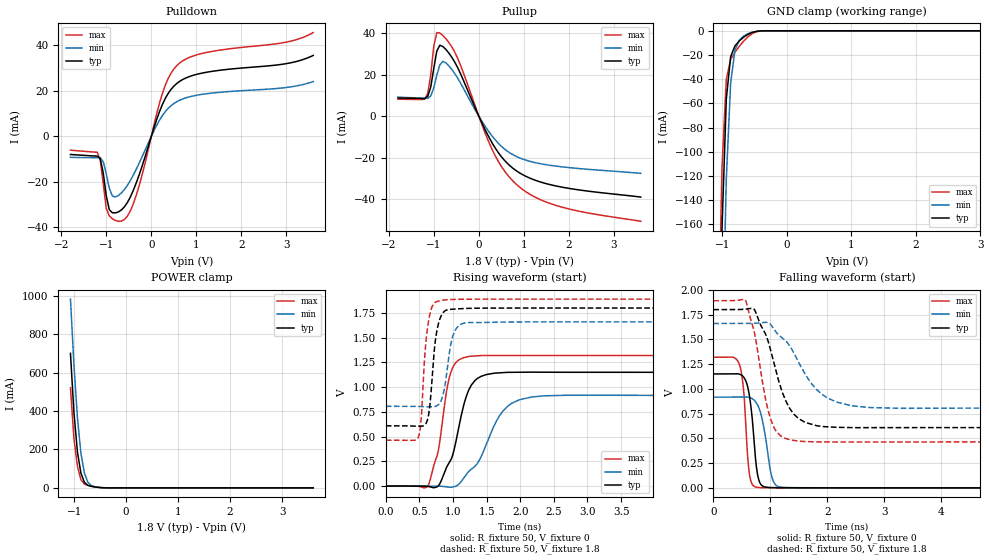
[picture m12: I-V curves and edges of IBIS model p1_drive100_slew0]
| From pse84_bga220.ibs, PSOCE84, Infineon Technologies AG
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[Model] p1_drive100_slew0
Model_type I/O
Polarity  Non-Inverting
Enable   Active-High
Vinl  =  0.54
Vinh  =  1.26
Vmeas =  0.9
Cref  =  15pF
| Capacitance   typ   min   max
C_comp   1.187163e-12   1.148471e-12   1.233738e-12
| Variables   typ   min   max
[GND Clamp Reference]   0   0   0
[POWER Clamp Reference]   1.8   1.66   1.89
[Pulldown Reference]   0   0   0
[Pullup Reference]   1.8   1.66   1.89
[Temperature Range]   25   125   -40
[Voltage Range]   1.8   1.66   1.89
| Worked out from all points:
|   slope of the pulldown table from 0 to 0.27 V, typ, clamps not added: 18 ohm
|   slope of the pullup table from 0 to 0.27 V, typ, clamps not added: 22.7 ohm
|   GND clamp passes 1 mA (typ) near -0.51 V on its own axis
|   POWER clamp passes 1 mA (typ) near -0.47 V on its own axis
|   rising waveform, R_fixture 50, V_fixture 0: 20-80 % time 266ps typ, 419ps min, 189ps max; typ from 0 V to 1.15 V
|   rising waveform, R_fixture 50, V_fixture 1.8: 20-80 % time 97.2ps typ, 117ps min, 87.9ps max; typ from 0.609 V to 1.8 V
|   falling waveform, R_fixture 50, V_fixture 0: 20-80 % time 116ps typ, 158ps min, 91.1ps max; typ from 1.15 V to 0 V
|   falling waveform, R_fixture 50, V_fixture 1.8: 20-80 % time 392ps typ, 582ps min, 272ps max; typ from 1.8 V to 0.609 V
[GND Clamp]
| Voltage   I(typ)   I(min)   I(max)
-1.137V   -618.8mA   -753.3mA   -532.4mA
-1.07V    -360.9mA   -497.6mA   -281.1mA
-1.003V   -163.7mA   -277.5mA   -113mA
-936.6mV  -56.21mA   -122.2mA   -40.06mA
-869.7mV  -21.33mA   -43.29mA   -23.66mA
-802.8mV  -12.5mA    -15.96mA   -17.71mA
-735.9mV  -8.345mA   -7.674mA   -12.88mA
-669mV    -5.267mA   -4.349mA   -8.574mA
-535.2mV  -1.314mA   -1.207mA   -2.328mA
-401.4mV  -73.55uA   -132.2uA   -119.3uA
3.6V      0A         0A         0A
[POWER Clamp]
| Voltage   I(typ)   I(min)   I(max)
-1.07V    700.8mA    983.4mA    521.5mA
-1.003V   391.6mA    640.4mA    255.8mA
-936.6mV  187.6mA    365.2mA    112.5mA
-869.7mV  77.29mA    181mA      42.73mA
-802.8mV  28.91mA    77.52mA    19.98mA
-735.9mV  13.13mA    29.19mA    13.35mA
-669mV    7.755mA    11.55mA    8.955mA
-535.2mV  2.356mA    2.862mA    2.667mA
-334.5mV  34.33uA    127.4uA    15.58uA
3.6V      0A         0A         0A
[Pullup]
| Voltage   I(typ)   I(min)   I(max)
-1.8V     8.819mA    9.225mA    8.256mA
-1.204V   8.594mA    8.734mA    8.362mA
-1.07V    14.25mA    9.887mA    20.21mA
-1.003V   23.19mA    13.79mA    33.91mA
-936.6mV  31.46mA    19.78mA    40.38mA
-869.7mV  34.26mA    24.82mA    40.18mA
-735.9mV  32.26mA    25.83mA    37.45mA
-468.3mV  23.29mA    18.27mA    27.8mA
310.3mV   -13.41mA   -9.935mA   -16.71mA
806.9mV   -25.84mA   -19.05mA   -32.25mA
1.738V    -33.65mA   -24.05mA   -43.07mA
3.6V      -38.9mA    -27.47mA   -50.57mA
[Pulldown]
| Voltage   I(typ)   I(min)   I(max)
-1.8V     -8.09mA    -9.336mA   -6.18mA
-1.204V   -8.819mA   -9.493mA   -7.128mA
-1.137V   -9.825mA   -9.491mA   -10.67mA
-1.003V   -26.32mA   -16.67mA   -31.9mA
-936.6mV  -32.37mA   -22.89mA   -35.09mA
-869.7mV  -33.73mA   -26.29mA   -36.32mA
-669mV    -32.52mA   -25.02mA   -37.41mA
-401.4mV  -23.83mA   -17.14mA   -29.77mA
248.3mV   14.08mA    9.149mA    19.02mA
558.6mV   23.07mA    15.08mA    30.9mA
1.117V    27.69mA    18.36mA    36.34mA
3.6V      35.52mA    24.01mA    45.58mA
[Ramp]
dV/dt_r   0.690092/0.265717n  0.54975/0.418773n  0.791747/0.1894n
dV/dt_f   0.714838/0.391602n  0.512302/0.581669n  0.855898/0.272071n
R_load = 50
[Rising Waveform]
R_fixture = 50
V_fixture = 0
V_fixture_min = 0
V_fixture_max = 0
| Time   V(typ)   V(min)   V(max)
0s        14.93nV    1.041uV    5.447nV
609.9ps   -2.759mV   823.6nV    -10.2mV
786.7ps   6.51mV     -1.184mV   381.1mV
898.1ps   181.7mV    -7.774mV   938mV
983.7ps   291.3mV    -11.34mV   1.182V
1.203ns   919.2mV    123.2mV    1.305V
1.395ns   1.101V     267.5mV    1.319V
1.81ns    1.15V      805.9mV    1.32V
2.678ns   1.15V      917.8mV    1.319V
50ns      1.15V      916.3mV    1.32V
[Rising Waveform]
R_fixture = 50
V_fixture = 1.8
V_fixture_min = 1.66
V_fixture_max = 1.89
| Time   V(typ)   V(min)   V(max)
0s        608.6mV    806.2mV    463.5mV
486.4ps   605mV      804.5mV    500.3mV
525ps     605mV      803.2mV    669.8mV
600.4ps   635.9mV    801.8mV    1.487V
765.6ps   1.592V     813.1mV    1.867V
862.2ps   1.761V     953.2mV    1.881V
967.8ps   1.787V     1.437V     1.886V
1.147ns   1.795V     1.644V     1.889V
1.907ns   1.8V       1.659V     1.89V
50ns      1.8V       1.66V      1.89V
[Falling Waveform]
R_fixture = 50
V_fixture = 0
V_fixture_min = 0
V_fixture_max = 0
| Time   V(typ)   V(min)   V(max)
0s        1.15V      916.3mV    1.32V
448.9ps   1.149V     916.6mV    1.259V
522.2ps   1.125V     918mV      1.038V
570.5ps   1.08V      917.9mV    626mV
649ps     869.9mV    909.8mV    90.82mV
750.4ps   240.4mV    863.9mV    6.796mV
801.1ps   75.33mV    807.3mV    2.825mV
1.041ns   2.205mV    86.26mV    804.9uV
1.284ns   813.2uV    3.524mV    336.9uV
50ns      14.89nV    1.093uV    5.439nV
[Falling Waveform]
R_fixture = 50
V_fixture = 1.8
V_fixture_min = 1.66
V_fixture_max = 1.89
| Time   V(typ)   V(min)   V(max)
0s        1.8V       1.66V      1.89V
551.8ps   1.804V     1.66V      1.902V
719.6ps   1.802V     1.662V     1.572V
918.9ps   1.549V     1.672V     891mV
1.065ns   1.258V     1.602V     608.6mV
1.275ns   874.6mV    1.483V     498.3mV
1.59ns    668.4mV    1.172V     468.1mV
2.164ns   611.5mV    866mV      463.3mV
3.27ns    608.2mV    803.1mV    463.6mV
50ns      608.6mV    806.2mV    463.5mV
